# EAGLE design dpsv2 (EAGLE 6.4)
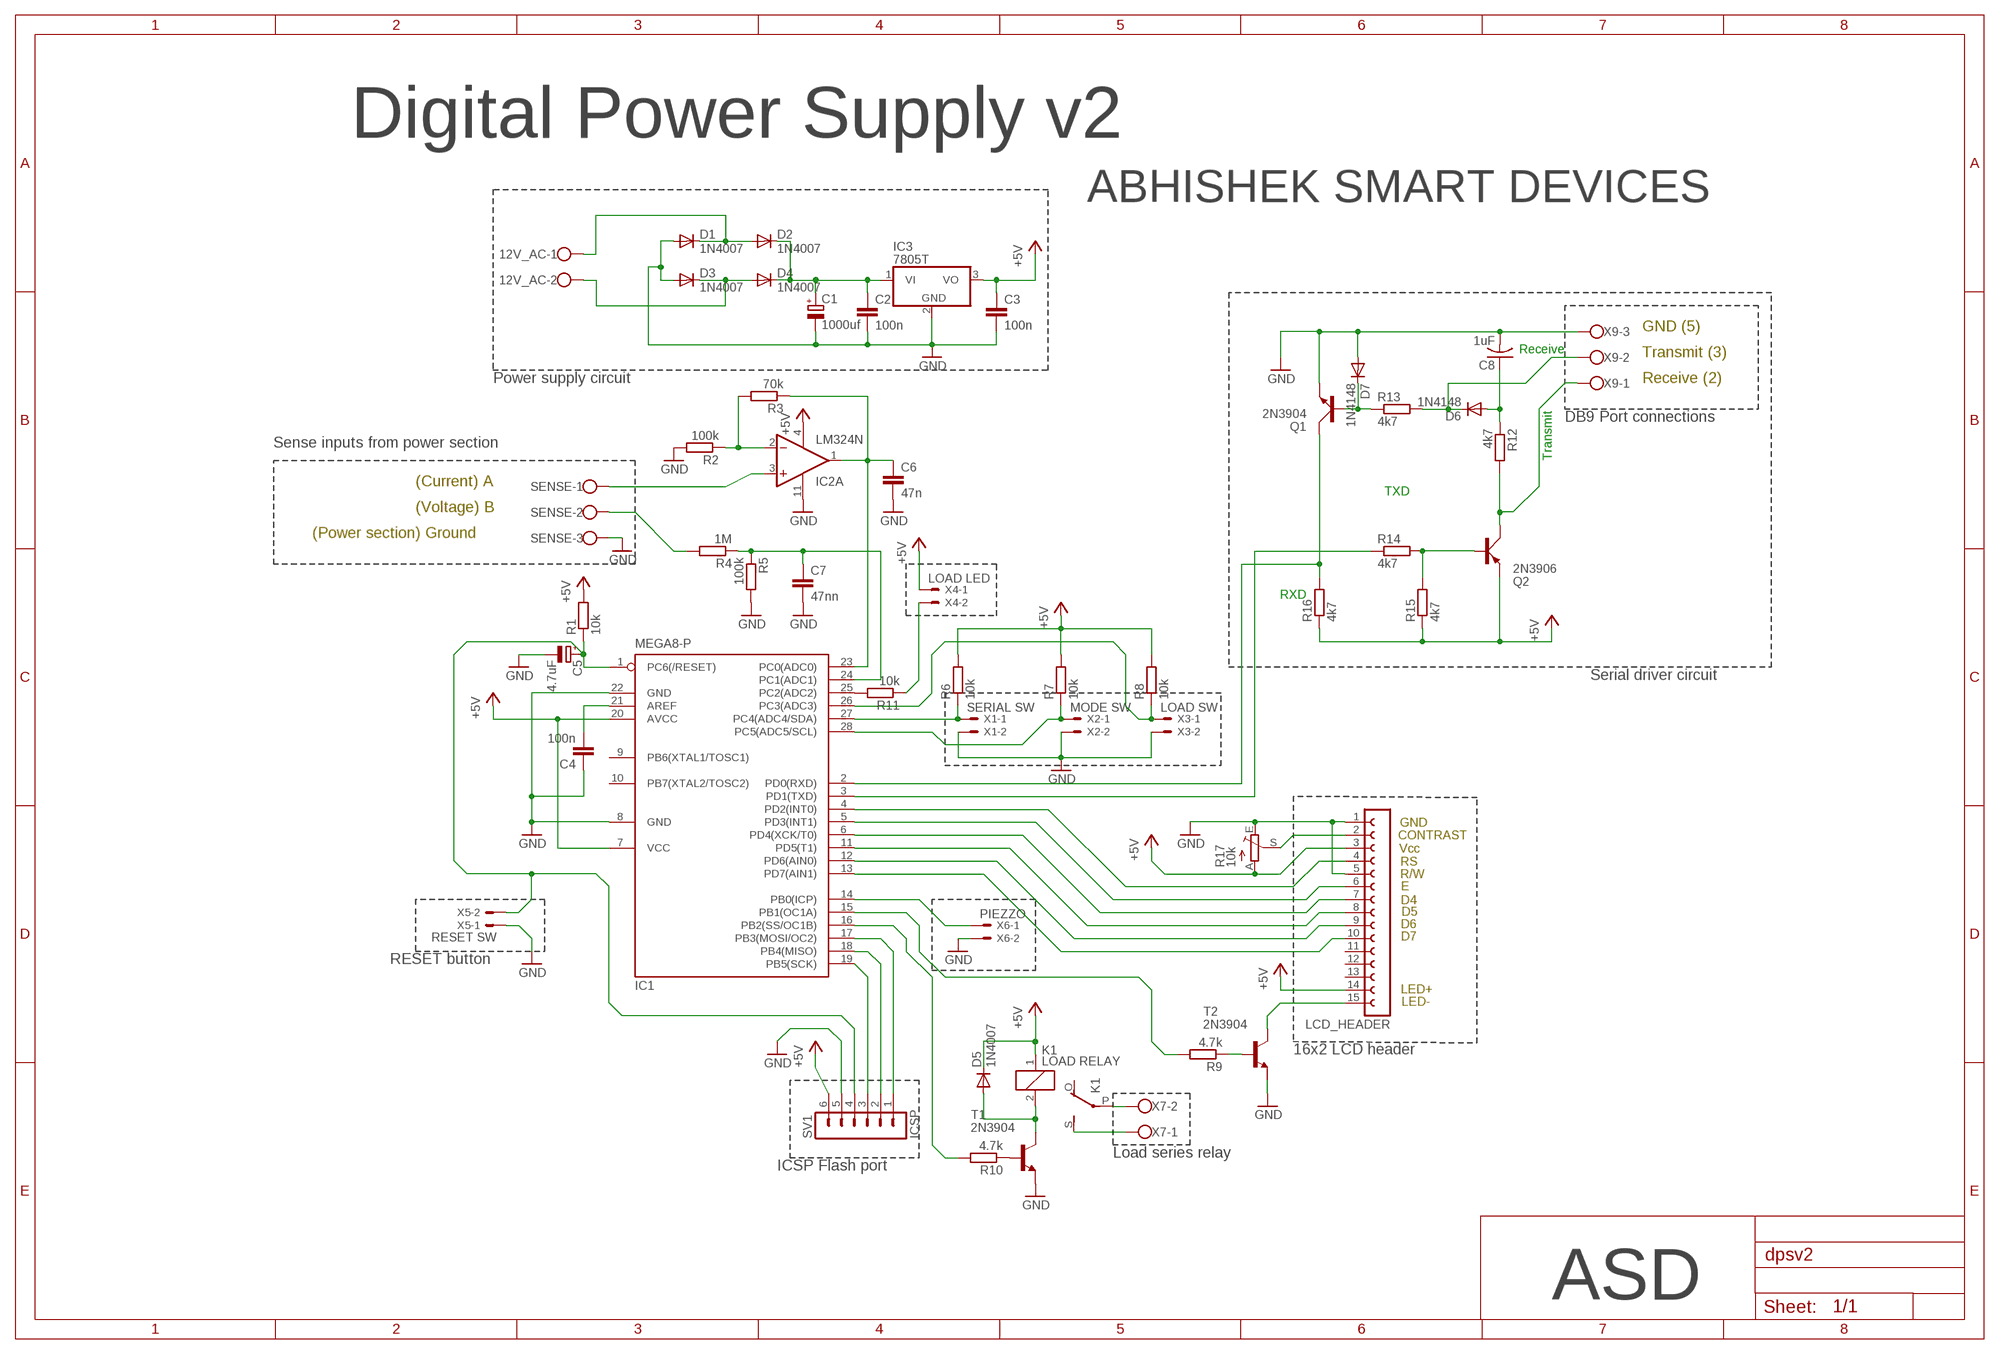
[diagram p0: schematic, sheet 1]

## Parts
12V_AC  W237-102  [W237-102]
C1  1000uf  CPOL-EUE5-13  [E5-13]
C2  100n  C-EU102-054X133  [C102-054X133]
C3  100n  C-EU102-054X133  [C102-054X133]
C4  100n  C-EU102-054X133  [C102-054X133]
C5  4.7uF  CPOL-EUE2.5-7  [E2,5-7]
C6  47n  C-EU050-025X075  [C050-025X075]
C7  47nn  C-EU050-025X075  [C050-025X075]
C8  1uF  C-US025-040X050  [C025-040X050]
D1  1N4007  DIODE-DO07  [DO07]
D2  1N4007  DIODE-DO07  [DO07]
D3  1N4007  DIODE-DO07  [DO07]
D4  1N4007  DIODE-DO07  [DO07]
D5  1N4007  DIODE-DO07  [DO07]
D6  1N4148  [DO35-10]
D7  1N4148  [DO35-10]
IC1  MEGA8-P  [DIL28-3]
IC2  LM324N  [DIL14]
IC3  7805T  [TO220H]
K1  LOAD RELAY  G5L  [G5LE]
LCD_HEADER  FE15-1  [FE15]
Q1  2N3904  [TO92D]
Q2  2N3906  [TO92D]
R1  10k  R-EU_0309/12  [0309/12]
R2  100k  R-EU_0309/12  [0309/12]
R3  70k  R-EU_0309/12  [0309/12]
R4  1M  R-EU_0309/12  [0309/12]
R5  100k  R-EU_0309/12  [0309/12]
R6  10k  R-EU_0309/12  [0309/12]
R7  10k  R-EU_0309/12  [0309/12]
R8  10k  R-EU_0309/12  [0309/12]
R9  4.7k  R-EU_0309/12  [0309/12]
R10  4.7k  R-EU_0309/12  [0309/12]
R11  10k  R-EU_0309/12  [0309/12]
R12  4k7  R-EU_0309/12  [0309/12]
R13  4k7  R-EU_0309/12  [0309/12]
R14  4k7  R-EU_0309/12  [0309/12]
R15  4k7  R-EU_0309/12  [0309/12]
R16  4k7  R-EU_0309/12  [0309/12]
R17  10k  TRIM_EU-B25X  [B25X]
SENSE  W237-103  [W237-103]
SV1  ICSP  MA06-1  [MA06-1]
T1  2N3904  BC548-NPN-TO92-CBE  [TO92-CBE]
T2  2N3904  BC548-NPN-TO92-CBE  [TO92-CBE]
X1  SERIAL SW  22-23-2021  [22-23-2021]
X2  MODE SW  22-23-2021  [22-23-2021]
X3  LOAD SW  22-23-2021  [22-23-2021]
X4  LOAD LED  22-23-2021  [22-23-2021]
X5  RESET SW  22-23-2021  [22-23-2021]
X6  PIEZZO  22-23-2021  [22-23-2021]
X7  W237-102  [W237-102]
X9  W237-103  [W237-103]

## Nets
+5V: C3.1 D5.C IC1.7(VCC) IC1.20(AVCC) IC2.4(P:V+) IC3.3(VO) K1.1 LCD_HEADER.3 LCD_HEADER.14 Q2.E R1.2 R6.2 R7.2 R8.2 R15.1 R16.1 R17.A SV1.6 X4.1
GND: C1.- C2.2 C3.2 C4.1 C5.- C6.2 C7.2 C8.2 D1.A D3.A D7.A IC1.8(GND) IC1.22(GND) IC2.11(P:V-) IC3.2(GND) LCD_HEADER.1 LCD_HEADER.5 Q1.E R2.2 R5.2 R17.E SENSE.3 SV1.5 T1.E T2.E X1.2 X2.2 X3.2 X5.1 X6.2 X9.3
N$1: C6.1 IC1.23(PC0(ADC0)) IC2.1(A:OUT) R3.1
N$2: 12V_AC.1 D1.C D2.A
N$3: 12V_AC.2 D3.C D4.A
N$4: C1.+ C2.1 D2.C D4.C IC3.1(VI)
N$5: IC2.3(A:+IN) SENSE.1
N$6: R4.2 SENSE.2
N$7: C4.2 IC1.21(AREF)
N$8: C7.1 IC1.24(PC1(ADC1)) R4.1 R5.1
N$9: C5.+ IC1.1(PC6(/RESET)) R1.1 SV1.4 X5.2
N$10: IC2.2(A:-IN) R2.1 R3.2
N$11: IC1.27(PC4(ADC4/SDA)) R6.1 X1.1
N$12: IC1.28(PC5(ADC5/SCL)) R7.1 X2.1
N$13: IC1.26(PC3(ADC3)) R8.1 X3.1
N$14: LCD_HEADER.15 T2.C
N$15: IC1.15(PB1(OC1A)) R9.2
N$16: IC1.16(PB2(SS/OC1B)) R10.2
N$17: R9.1 T2.B
N$18: R10.1 T1.B
N$19: D5.A K1.2 T1.C
N$20: IC1.14(PB0(ICP)) X6.1
N$21: K1.P(2:P) X7.2
N$22: IC1.25(PC2(ADC2)) R11.2
N$23: R11.1 X4.2
N$24: K1.S(2:S) X7.1
N$25: IC1.17(PB3(MOSI/OC2)) SV1.1
N$26: IC1.18(PB4(MISO)) SV1.2
N$27: IC1.19(PB5(SCK)) SV1.3
N$28: IC1.2(PD0(RXD)) Q1.C R16.2
N$29: Q2.B R14.2 R15.2
N$30: C8.1 D6.A R12.1
N$31: Q2.C R12.2 X9.1
N$32: D7.C Q1.B R13.1
N$33: D6.C R13.2 X9.2
N$34: IC1.5(PD3(INT1)) LCD_HEADER.6
N$35: IC1.3(PD1(TXD)) R14.1
N$36: LCD_HEADER.2 R17.S
N$37: IC1.6(PD4(XCK/T0)) LCD_HEADER.7
N$38: IC1.11(PD5(T1)) LCD_HEADER.8
N$39: IC1.12(PD6(AIN0)) LCD_HEADER.9
N$40: IC1.4(PD2(INT0)) LCD_HEADER.4
N$41: IC1.13(PD7(AIN1)) LCD_HEADER.10
Unconnected: IC1.9(PB6(XTAL1/TOSC1)) IC1.10(PB7(XTAL2/TOSC2)) IC2.5(B:+IN) IC2.6(B:-IN) IC2.7(B:OUT) IC2.8(C:OUT) IC2.9(C:-IN) IC2.10(C:+IN) IC2.12(D:+IN) IC2.13(D:-IN) IC2.14(D:OUT) K1.O(2:O) LCD_HEADER.11 LCD_HEADER.12 LCD_HEADER.13

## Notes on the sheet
- Digital Power Supply v2
- ABHISHEK SMART DEVICES
- GND (5)
- Receive
- Transmit (3)
- Power supply circuit | Receive (2)
- DB9 Port connections
- Sense inputs from power section
- Transmit
- (Current) A | TXD
- (Voltage) B
- (Power section) Ground
- RXD
- Serial driver circuit
- GND
- CONTRAST
- Vcc
- RS
- R/W
- E
- D4
- D5
- D6
- D7
- RESET button
- LED+
- LED-
- 16x2 LCD header
- Load series relay
- ICSP Flash port
- ASD

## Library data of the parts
12V_AC X7 = con-wago-500:W237-102: WAGO SCREW CLAMP; MPN: 237-102; OC_FARNELL: unknown; OC_NEWARK: 70K9898
C1 C5 = resistor:CPOL-EU: POLARIZED CAPACITOR, European symbol
C2-C4 C6 C7 = resistor:C-EU: CAPACITOR, European symbol
C8 = resistor:C-US: CAPACITOR, American symbol
D1-D5 = diode:DIODE-: DIODE
D6 D7 = diode:1N4148: DIODE
IC1 = atmel:MEGA8-P: MICROCONTROLLER 8 Kbytes FLASH, 1 kbytes SRAM, 512 bytes EEPROM, USART, 4-channel 10 bit ADC, 2-channel 8 bit ADC Pin compatible with Atmega48, ATMega88, ATMega168 Source: avr.lbr; OC_FARNELL: unknown; OC_NEWARK: unknown
IC2 = linear:LM324: OP AMP
IC3 = linear:78*: Positive VOLTAGE REGULATOR Source: http://cache.national.com/ds/LM/LM78L05.pdf http://www.fairchildsemi.com/ds/LM/LM7805.pdf
K1 = relay:G5L: RELAY 1 x switch, 10 A/120 V AC, 8 A/30 V ADC, Omron; OC_FARNELL: unknown; OC_NEWARK: unknown
LCD_HEADER = con-lsta:FE15-1: FEMALE HEADER; OC_FARNELL: unknown; OC_NEWARK: unknown
Q1 = transistor-small-signal:2N3904: NPN TRANSISTOR
Q2 = transistor-small-signal:2N3906: PNP TRANSISTOR
R1-R16 = resistor:R-EU_: RESISTOR, European symbol
R17 = pot:TRIM_EU-: POTENTIOMETER
SENSE X9 = con-wago-500:W237-103: WAGO SCREW CLAMP; MPN: 237-103; OC_FARNELL: unknown; OC_NEWARK: 18M7116
SV1 = con-lstb:MA06-1: PIN HEADER; OC_FARNELL: unknown; OC_NEWARK: unknown
T1 T2 = transistor:*-NPN-: NPN Transistror BF959 corrected 2008.03.06
X1-X6 = con-molex:22-23-2021: .100" (2.54mm) Center Header - 2 Pin; MF: MOLEX; MPN: 22-23-2021; OC_FARNELL: 1462926; OC_NEWARK: 25C3832

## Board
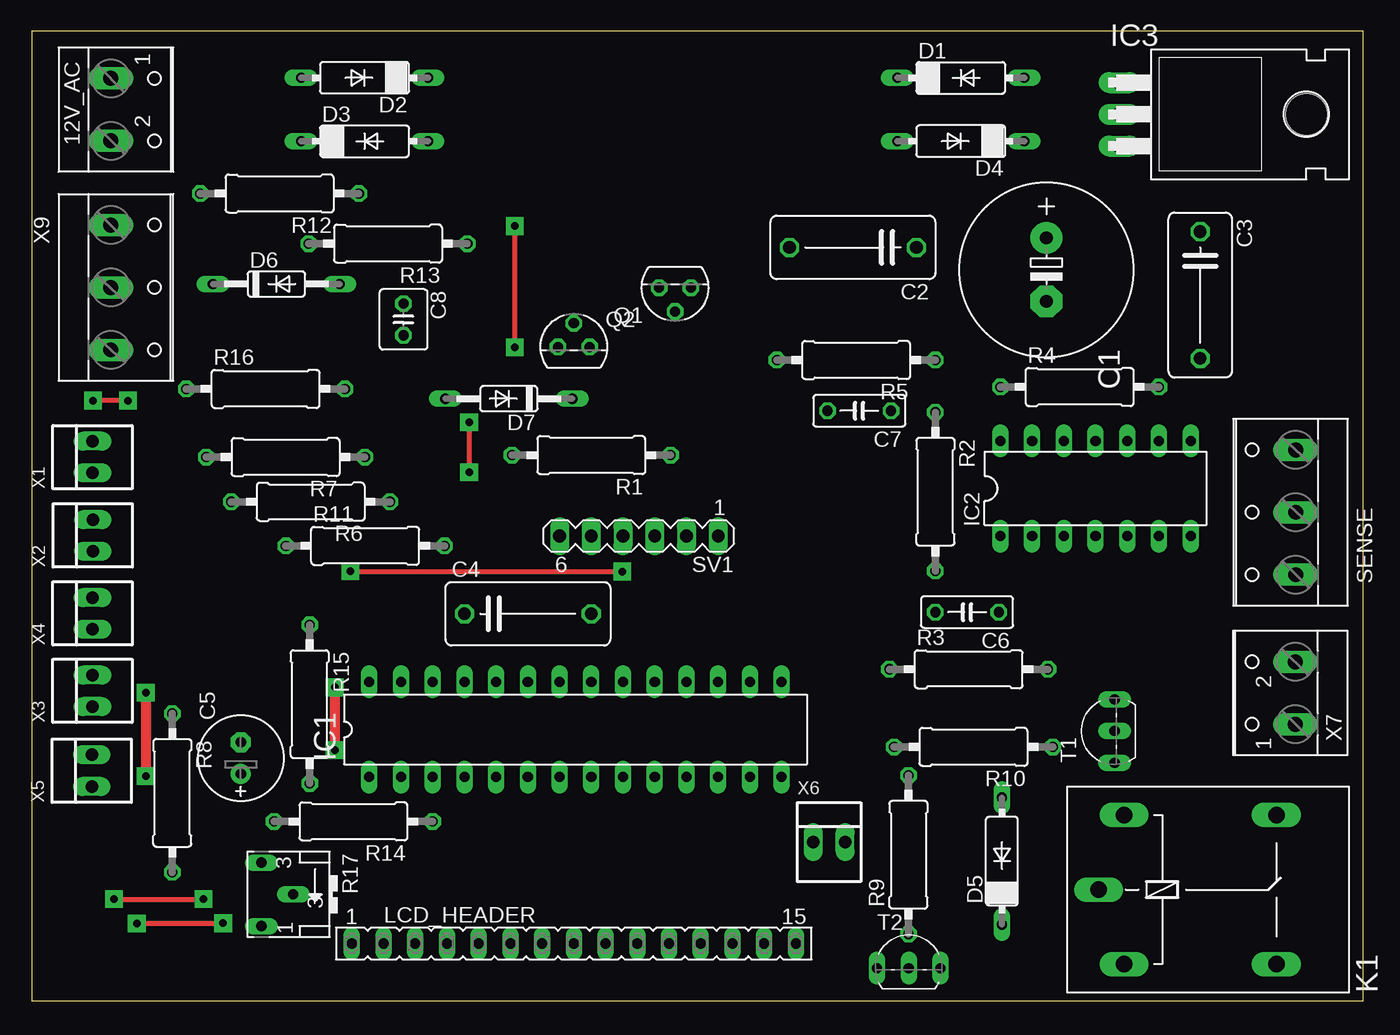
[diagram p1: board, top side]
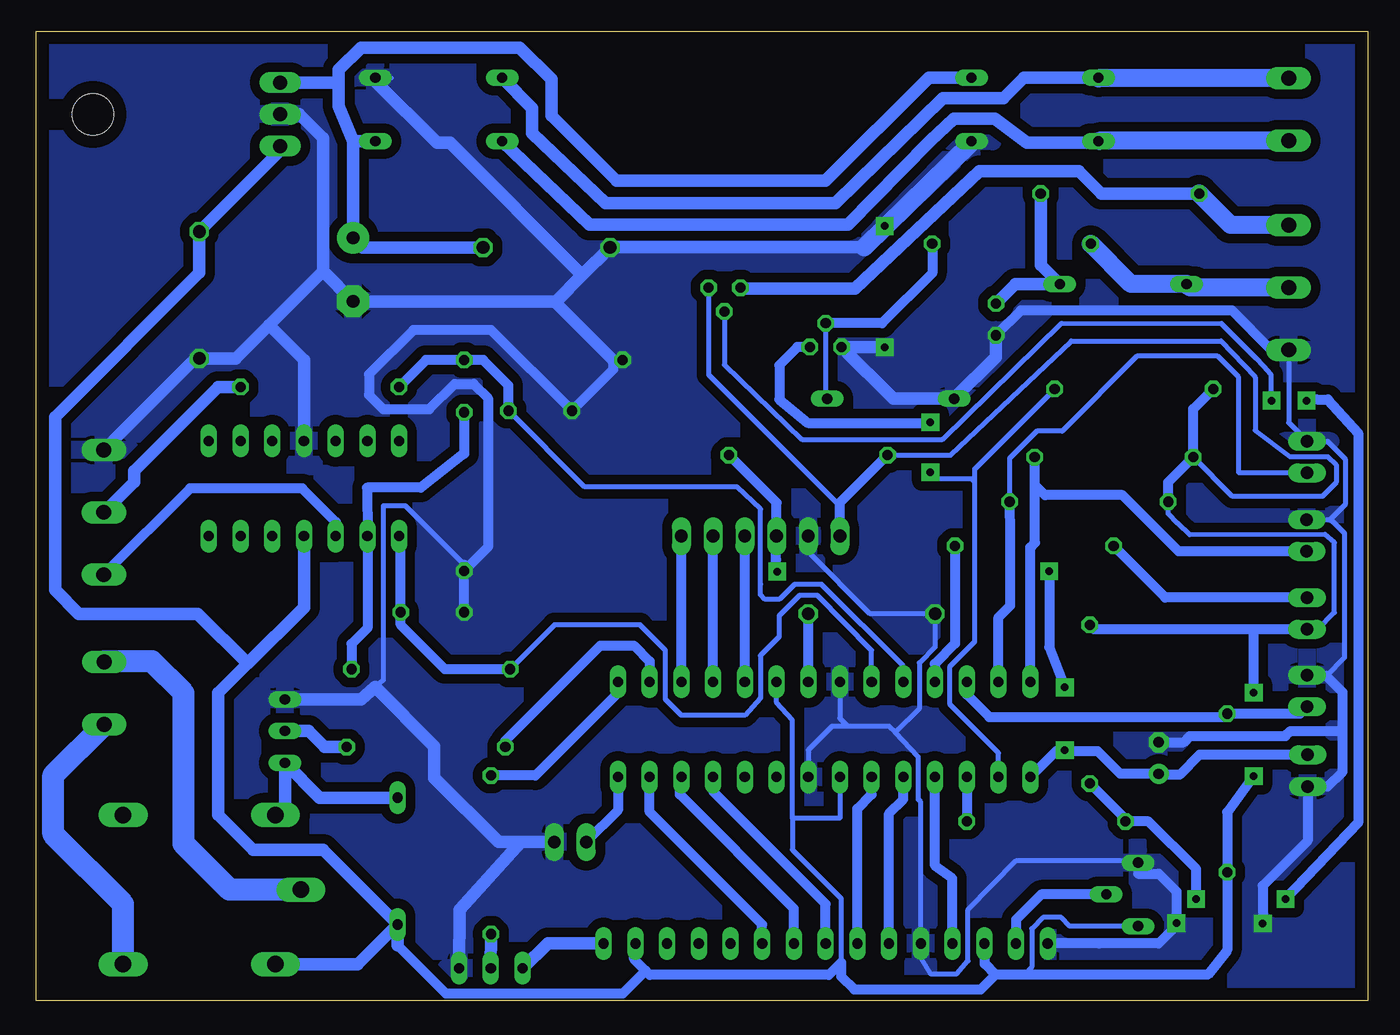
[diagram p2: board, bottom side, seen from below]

Size 106.66 x 77.65 mm. Coordinates in mm from the lower left corner, seen from the top.
Outline: 0,0 106.66,0 106.66,77.65 0,77.65 0,0
Copper layers (1*16): Top 0.035mm / dielectric 1.5mm / Bottom 0.035mm
Design rules "default *": minimum track width 10mil, minimum drill 24mil, track to track 30mil, track to pad 30mil, pad to pad 8mil, via to via 8mil, smd to smd 8mil, copper to edge 40mil, drill to drill 8mil, minimum pad ring 10mil, minimum via ring 8mil, stop-mask expansion 4mil, vias tented up to drill 0mil, thermal gap 10mil

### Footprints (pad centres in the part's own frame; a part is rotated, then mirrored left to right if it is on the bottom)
W237-102 = drill 1.194 long: 1 -2.5,-1.27; 2 2.5,-1.27
E5-13 = drill 1.016 pad 2.54: + -2.54,0 | drill 1.016 pad 2.54 octagon: - 2.54,0
C102-054X133 = drill 1.016 octagon: 1 -5.08,0; 2 5.08,0
E2,5-7 = drill 0.813 pad 1.6: + -1.27,0 | drill 0.813 pad 1.6 octagon: - 1.27,0
C050-025X075 = drill 0.813 octagon: 1 -2.54,0; 2 2.54,0
C025-040X050 = drill 0.813 octagon: 1 -1.27,0; 2 1.27,0
DO07 = drill 0.813 long: A 5.08,0; C -5.08,0
DO35-10 = drill 0.813 long: A 5.08,0; C -5.08,0
DIL28-3 = drill 0.813 long: 1 -16.51,-3.81; 2 -13.97,-3.81; 3 -11.43,-3.81; 4 -8.89,-3.81; 5 -6.35,-3.81; 6 -3.81,-3.81; 7 -1.27,-3.81; 8 1.27,-3.81; 9 3.81,-3.81; 10 6.35,-3.81; 11 8.89,-3.81; 12 11.43,-3.81; 13 13.97,-3.81; 14 16.51,-3.81; 15 16.51,3.81; 16 13.97,3.81; 17 11.43,3.81; 18 8.89,3.81; 19 6.35,3.81; 20 3.81,3.81; 21 1.27,3.81; 22 -1.27,3.81; 23 -3.81,3.81; 24 -6.35,3.81; 25 -8.89,3.81; 26 -11.43,3.81; 27 -13.97,3.81; 28 -16.51,3.81
DIL14 = drill 0.813 long: 1 -7.62,-3.81; 2 -5.08,-3.81; 3 -2.54,-3.81; 4 0,-3.81; 5 2.54,-3.81; 6 5.08,-3.81; 7 7.62,-3.81; 8 7.62,3.81; 9 5.08,3.81; 10 2.54,3.81; 11 0,3.81; 12 -2.54,3.81; 13 -5.08,3.81; 14 -7.62,3.81
TO220H = drill 1.118 long: 1 -2.54,-10.16; 2 0,-10.16; 3 2.54,-10.16 | hole 3.302: 0,4.826
G5LE = drill 1.321 long: 1 -7.493,-5.969; 2 -7.493,5.969; O 4.699,5.969; P -9.525,0; S 4.699,-5.969
FE15 = drill 0.813 long: 1 -17.78,0; 2 -15.24,0; 3 -12.7,0; 4 -10.16,0; 5 -7.62,0; 6 -5.08,0; 7 -2.54,0; 8 0,0; 9 2.54,0; 10 5.08,0; 11 7.62,0; 12 10.16,0; 13 12.7,0; 14 15.24,0; 15 17.78,0
TO92D = drill 0.813 octagon: B 0,1.905; C 1.27,0; E -1.27,0
0309/12 = drill 0.813 octagon: 1 -6.35,0; 2 6.35,0
B25X = drill 0.813 long: A 2.54,-1.905; E -2.54,-1.905; S 0,0.635
W237-103 = drill 1.194 long: 1 -5,-1.29; 2 0,-1.29; 3 5,-1.29
MA06-1 = drill 1.016 long: 1 -6.35,0; 2 -3.81,0; 3 -1.27,0; 4 1.27,0; 5 3.81,0; 6 6.35,0
TO92-CBE = drill 0.813 long: B 0,0; C -2.54,0; E 2.54,0
22-23-2021 = drill 1 long: 1 -1.27,0; 2 1.27,0

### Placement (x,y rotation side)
12V_AC  7.62,71.37 270 top
C1  81.28,58.55 270 top
C2  65.79,60.33 180 top
C3  93.6,56.52 270 top
C4  39.75,30.99 0 top
C5  16.76,19.43 90 top
C6  74.93,31.12 180 top
C7  66.29,47.24 180 top
C8  29.79,54.56 270 top
D1  74.42,73.91 0 top
D2  26.67,73.91 180 top
D3  26.67,68.83 0 top
D4  74.42,68.83 180 top
D5  77.72,11.18 90 top
D6  19.61,57.4 0 top
D7  38.23,48.21 180 top
IC1  43.56,21.72 0 top
IC2  85.22,41.02 0 top
IC3  97.28,70.99 270 top
K1  95,8.89 0 top
LCD_HEADER  43.43,4.57 0 top
Q1  43.43,52.35 0 top
Q2  51.54,57.1 180 top
R1  44.83,43.69 180 top
R2  72.39,40.77 270 top
R3  75.06,26.54 0 top
R4  83.95,49.15 0 top
R5  66.04,51.31 180 top
R6  22.35,39.95 180 top
R7  20.35,43.54 180 top
R8  11.28,16.64 270 top
R9  70.23,11.68 90 top
R10  75.44,20.32 180 top
R11  26.72,36.42 0 top
R12  19.86,64.64 180 top
R13  28.55,60.63 180 top
R14  25.78,14.35 180 top
R15  22.28,23.75 270 top
R16  18.75,49 0 top
R17  20.32,8.51 270 top
SENSE  99.95,39.12 90 top
SV1  48.64,37.21 180 top
T1  86.74,21.59 90 top
T2  70.26,2.59 0 top
X1  4.88,43.54 90 top
X2  4.9,37.26 90 top
X3  4.88,24.82 90 top
X4  4.88,31.01 90 top
X5  4.83,18.41 90 top
X6  63.88,12.7 0 top
X7  99.95,24.64 90 top
X9  7.65,57.12 270 top

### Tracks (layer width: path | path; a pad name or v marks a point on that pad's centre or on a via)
+5V  (via drill 0.6 pad 1.42)
  Top 0.813: v9.14,24.66 v9.14,17.98
  Bottom 0.406: IC3.3 87.12,68.07 | IC1.7 42.29,14.61 46.1,14.61 | 46.1,14.61 46.1,22.48 47.37,23.88 IC1.20 | 42.29,39.88 42.29,39.62 52.81,50.14 Q2.E | 21.92,29.74 R15.1 | X4.1 4.04,29.74 2.69,31.09 2.69,36.68 3.45,37.34 14.27,37.31 15.21,38.23 16,39.01 R6.2 | R1.2 33.43,43.69 23.77,52.83 11.79,52.83 9.04,49.94 9.04,45.67 6.25,43.56 3.2,43.56 2.54,42.93 2.54,41.5 3.66,40.39 10.85,40.39 R7.2 | 30.68,4.52 LCD_HEADER.3 | R17.A 23.88,5.97 24.56,6.66 26.03,6.66 26.92,5.77 26.92,2.69 27.53,2.08 | 46.1,14.61 46.1,12.09 42.19,8.18 42.19,3.05 | 58.78,4.47 LCD_HEADER.14
  Bottom 0.813: SV1.6 42.29,39.62 | 42.29,39.88 R1.2 | R16.1 13.99,47.4 R7.2 16,41.53 R6.2 | X4.1 9.14,29.74 | 9.14,29.74 21.92,29.74 | v9.14,17.98 11.28,15.09 R8.2 11.28,4.04 12.83,2.08 27.53,2.08 29.82,2.08 | v9.14,24.66 9.14,29.74 | 30.68,4.52 30.68,2.95 29.82,2.08 | 57.85,2.4 57.51,2.06 43.18,2.06 42.19,3.05 42.19,1.93 41.15,0.89 31.01,0.89 29.82,2.08 | 57.85,2.4 58.78,3.33 58.78,4.47 | 77.72,4.45 73.86,0.58 59.66,0.58 57.85,2.4
  Bottom 1.016: 87.12,68.07 C3.1 93.6,58.29 105.16,46.74 105.16,32.89 103.25,30.99 93.73,30.99 89.73,26.99 | IC2.4 85.22,31.5 89.73,26.99 | 89.73,26.99 92.07,24.64 92.07,14.86 89.28,12.06 83.69,12.06 D5.C | K1.1 80.9,2.92 D5.C | D5.C 77.72,4.45
GND  (via drill 0.6 pad 1.42)
  Top 0.406: v8.43,6.17 v15.34,6.2 | v38.71,52.32 v38.71,62.04
  Bottom 0.406: 78.23,73.91 D1.A 79.5,73.66 | 65.15,56.01 65.02,56.01 | C3.2 93.92,51.44 | R5.2 60.45,51.31 | C6.2 R2.2 | 72.39,34.93 77.09,39.62 78.87,39.62 78.87,25.65 79.5,25.11 | 37.85,21.46 36.02,19.53 36.02,16.1 35.81,15.9 LCD_HEADER.5 35.81,3.4 35.05,2.16 32.92,2.16 32.03,3.17 32.03,7.29 28.14,11.23 18.59,11.23 R17.E | 37.85,21.46 38.35,21.97 41.66,21.97 | 41.66,21.97 42.93,21.97 44.83,20.07 IC1.8 | IC1.22 42.29,22.61 41.66,21.97 | SV1.5 44.83,35.94 39.88,30.99 C4.1 34.67,28.32 35.94,27.05 35.94,23.37 37.85,21.46 | 4.8,26.01 X3.2 | 3.05,38.51 1.83,39.73 1.83,43.38 3.25,44.81 X1.2 6.35,46.28 X9.3 | 3.05,38.51 4.88,38.51 X2.2 | 21.49,4.52 21.54,4.57 | 3.05,38.51 2.95,38.51 1.88,37.44 1.88,27.48 3.35,26.01 | 2.34,21.59 2.03,21.9 | D3.A 31.75,68.73 | 60.53,60.35 C2.2 | 38.84,52.35 v38.71,52.32 | 38.56,62.09 v38.71,62.04 39.63,61.11 39.73,61.11 40.34,60.5 40.34,60.35 | v15.34,6.2 15.34,5.99
  Bottom 0.813: 60.45,51.31 60.45,50.55 C7.2 70.23,53.72 76.45,53.72 80.01,50.16 80.01,48.51 78.87,47.37 75.18,47.37 73.15,49.4 71.63,49.4 70.48,48.26 70.48,36.32 R2.2 | C6.2 72.39,34.93 | R17.E 18.41,10.16 16.76,10.16 15.34,8.74 v15.34,6.2 | LCD_HEADER.1 21.54,4.57 16.76,4.57 15.34,5.99 | 4.8,26.01 3.35,26.01 2.03,24.69 2.03,21.9 2.03,18.34 3.23,17.15 X5.1 4.83,12.8 8.43,9.2 v8.43,6.17 | C5.- 14.76,20.7 14.27,21.18 6.6,21.18 6.2,21.59 2.34,21.59 | X9.3 7.72,52.12 10.87,55.27 27.81,55.27 C8.2
  Bottom 1.016: IC3.2 85.6,70.99 83.69,69.09 83.69,58.42 | 83.69,58.42 C1.- 65.15,56.01 60.45,51.31 | 65.02,56.01 62.93,58.1 | 62.93,58.1 C2.2 | 79.5,73.66 74.55,68.71 73.53,68.71 62.93,58.1 | C3.2 90.68,51.44 88.01,54.1 | 88.01,54.1 83.69,58.42 | 93.92,51.44 SENSE.3 | X6.2 67.82,12.7 | 67.82,12.7 72.77,7.26 T2.E | IC2.11 85.22,51.31 88.01,54.1 | T1.E 80.64,24.13 79.5,25.11 74.78,20.38 74.78,17.83 69.65,12.7 67.82,12.7 | 40.34,60.35 60.53,60.35 | C8.2 29.79,51.56 D7.A 38.02,48.21 Q1.E 38.84,52.35
  Bottom 1.422: 31.75,68.73 40.34,60.35
  pour Bottom: -1.02,78.13 -1.02,-0.61 -0.33,-1.3 107.26,-1.3 108.92,0.36 108.92,77.32 106.73,79.5 0.36,79.5 -0.97,78.18
N$1
  Bottom 0.406: 77.47,37.08 IC2.1 | IC1.23 39.75,28.07 44.09,32.46 45.52,32.46 47.17,30.81 47.17,29.13 48.67,27.63 48.67,24.28 48.64,24.26 49.91,22.86 54.99,22.86 56.26,24.13 56.26,28.07 58.29,30.1 65.15,30.1 R3.1
  Bottom 0.813: 77.47,37.08 C6.1 77.47,30.1 73.91,26.54 R3.1
N$2
  Bottom 0.406: 21.59,73.87 D2.A
  Bottom 1.016: D2.A 27.56,73.91 29.21,72.26 34.04,72.26 42.65,63.88 61.06,63.88 66.93,69.47 66.93,71.5 D1.C
  Bottom 1.422: 12V_AC.1 21.59,73.87
N$3
  Bottom 0.406: 21.55,68.87 D3.C 21.72,68.71
  Bottom 1.016: 21.72,68.71 27.3,68.71 29.9,70.64 33.17,70.64 35.03,68.86 37.39,66.5 41.63,62.15 62.33,62.15 D4.A
  Bottom 1.422: 12V_AC.2 21.55,68.87
N$4
  Bottom 0.406: 82.55,73.53 82.42,73.66
  Bottom 1.016: 81.28,68.83 82.42,71.63 82.42,73.66 82.42,74.55 80.64,76.33 67.94,76.33 65.41,73.79 65.41,70.87 60.2,65.66 43.43,65.66 35.18,73.91 D2.C | 81.28,68.83 D4.C | IC3.1 82.55,73.53 | 81.28,68.83 C1.+ 80.52,60.33 C2.1
N$5
  Bottom 0.813: IC2.3 82.68,38.35 85.34,41.02 94.33,41.02 SENSE.1
N$6
  Bottom 1.016: R4.2 92.07,49.15 98.81,42.42 98.81,41.55 SENSE.2
N$7
  Bottom 0.813: IC1.21 C4.2
N$8
  Bottom 0.406: IC1.24 37.21,26.8 43.76,33.35 45.92,33.35 47.14,32.13 48.29,32.13 48.67,32.51 48.67,33.33 48.64,33.35 48.64,39.37 50.55,41.15 62.74,41.15 C7.1
  Bottom 0.813: R4.1 75.44,51.31 R5.1 70.87,51.31 68.83,49.28 C7.1
N$9  (via drill 0.6 pad 1.42)
  Top 0.406: v25.53,34.39 v47.32,34.37
  Top 0.813: v24.28,25.09 v24.28,20.07
  Bottom 0.406: 19.84,18.16 C5.+ 16.69,18.09 | 47.4,37.19 SV1.4 | v24.28,20.07 24.38,19.96
  Bottom 0.813: SV1.4 47.37,39.88 R1.1 | 19.84,18.16 21.64,19.96 24.38,19.96 24.99,19.96 IC1.1 | X5.2 13.49,19.69 15.09,18.09 16.69,18.09 | C5.+ 19.79,18.16 | v47.32,34.37 47.4,35.31 47.4,37.19 | v25.53,34.39 25.53,28.3 v24.28,25.09
N$10
  Bottom 0.813: R2.1 72.39,43.82 75.84,41.1 80.16,41.1 IC2.2 80.14,29.84 81.41,28.58 R3.2
N$11
  Bottom 0.406: X1.1 10.34,42.27 10.36,49.94 12.04,51.61 18.49,51.61 24.49,45.62 26.52,45.62 28.7,43.43 R6.1
  Bottom 0.813: IC1.27 29.59,30.71 28.65,31.65 28.65,38.18 R6.1
N$12
  Bottom 0.406: 26.67,43.51 R7.1
  Bottom 0.813: IC1.28 27.05,36.3 26.67,36.68 26.67,41.3 | 26.67,41.3 26.67,43.51 | X2.1 15.16,35.99 19.66,40.49 25.86,40.49 26.67,41.3
N$13
  Bottom 0.406: 11.2,22.71 R8.1
  Bottom 0.813: R8.1 5.44,22.99 X3.1 | IC1.26 32.13,24.51 30.33,22.71 11.2,22.71
N$14
  Bottom 1.016: LCD_HEADER.15 65.66,4.57 T2.C
N$15
  Bottom 0.813: IC1.15 60.07,24.64 66.67,18.03 R9.2
N$16
  Bottom 0.406: R10.2 69.09,20.83
  Bottom 0.813: 69.09,20.83 61.47,28.45 58.8,28.45 57.53,27.18 IC1.16
N$17
  Bottom 1.016: T2.B R9.1
N$18
  Bottom 1.016: R10.1 83.57,20.32 84.84,21.59 T1.B
N$19
  Bottom 1.016: K1.2 86.74,15.62 T1.C 83.95,16.26 D5.A
N$20
  Bottom 0.813: IC1.14 60.07,15.24 X6.1
N$21
  Bottom 0.406: 101.18,27.18 X7.2
  Bottom 1.778: K1.P 91.19,8.89 94.87,12.57 94.87,24.64 97.41,27.18 101.18,27.18
N$22
  Bottom 0.406: 34.7,25.55 IC1.25
  Bottom 0.813: R11.2 33.07,28.6 34.7,26.98 34.7,25.55
N$23
  Bottom 0.813: X4.2 16.23,32.28 R11.1
N$24
  Bottom 1.778: K1.S 99.69,7.75 105.28,13.34 105.28,18.07 X7.1
N$25
  Bottom 0.813: IC1.17 SV1.1
N$26
  Bottom 0.813: IC1.18 SV1.2
N$27
  Bottom 0.813: IC1.19 SV1.3
N$28  (via drill 0.6 pad 1.42)
  Top 0.406: v35.05,46.33 v35.05,42.32
  Bottom 0.406: IC1.2 29.59,19.84 33.48,23.72 33.48,26.77 31.5,28.75 31.5,41.55 | 31.5,41.55 31.5,42.6 R16.2 | 35.61,46.28 v35.05,46.33 | v35.05,42.32 34.54,41.81 31.75,41.81 31.5,41.55
  Bottom 0.813: Q1.C 45.7,52.35 47.14,50.9 47.14,48.16 44.86,46.28 35.61,46.28
N$29  (via drill 0.6 pad 1.42)
  Top 0.406: v7.72,48.06 v4.93,48.06 | v6.6,8.13 v13.77,8.13
  Bottom 0.406: R14.2 19.43,14.55 | Q2.B 51.54,50.93 45.31,44.96 34.09,44.96 24.54,54.25 11.73,54.23 8.99,51.49 8.38,50.83 7.77,50.14 7.77,48.11 v7.72,48.06 | v4.93,48.06 4.12,48.16
  Bottom 0.813: 19.43,14.55 R15.2 | 4.12,48.16 3.2,48.16 0.79,45.47 0.79,14.22 v6.6,8.13 | v13.77,8.13 13.77,10.54 17.58,14.35 R14.2
N$30
  Bottom 1.016: R12.1 26.21,58.93 D6.A 28.22,57.4 C8.1
N$31
  Bottom 0.406: 50.22,57.05 Q2.C
  Bottom 1.016: 50.22,57.05 41.07,57.05 31.14,66.45 23.14,66.45 21.34,64.64 R12.2
  Bottom 1.422: X9.1 10.99,62.12 R12.2
N$32
  Bottom 0.406: Q1.B 43.43,48.34 D7.C
  Bottom 0.813: R13.1 34.9,58.27 38.91,54.25 Q1.B
N$33
  Bottom 1.422: X9.2 14.25,57.12 D6.C 18.97,57.4 R13.2
N$34
  Bottom 0.813: LCD_HEADER.6 38.35,14.99 37.21,16.13 IC1.5
N$35
  Bottom 0.813: IC1.3 R14.1
N$36
  Bottom 0.813: R17.S 26.16,8.51 28.19,6.48 LCD_HEADER.2
N$37
  Bottom 0.813: LCD_HEADER.7 40.89,15.37 39.75,16.51 IC1.6
N$38
  Bottom 0.813: LCD_HEADER.8 43.43,7.75 52.45,16.76 IC1.11
N$39
  Bottom 0.406: 55.12,17.78 IC1.12
  Bottom 0.813: LCD_HEADER.9 45.97,7.37 55.12,16.51 55.12,17.78
N$40
  Bottom 0.813: LCD_HEADER.4 33.3,9.78 34.67,10.79 IC1.4
N$41
  Bottom 0.813: LCD_HEADER.10 48.51,6.1 57.53,15.11 IC1.13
